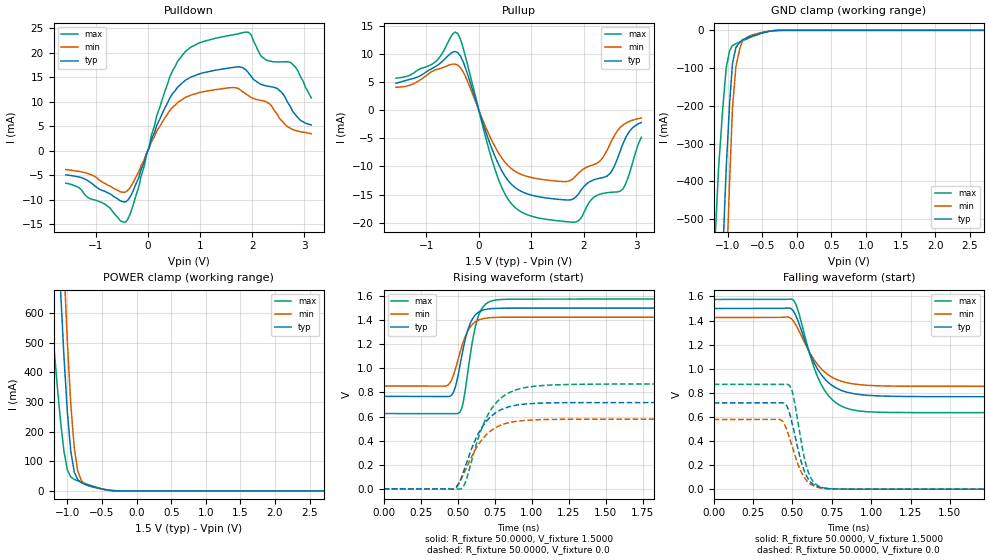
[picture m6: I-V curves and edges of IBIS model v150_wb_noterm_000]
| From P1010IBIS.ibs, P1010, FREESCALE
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[Model] v150_wb_noterm_000
|   Model v150_wb_noterm_000
| This model was characterised for following simulation conditions:
| External (pad) voltage:
|   - Typ: 1.5V,   - Min: 1.425V,   - Max: 1.575V
| Library cells for typ/min/max conditions are connected as defined below:
|  chip_pad - External Pad
|  ipp_do - Core Input
|  ipp_obe - Output Buffer Enable
|  esd_boost - vdd_io
|  gnd_io - gnd_io
|  vdd_d - vdd_d
|  vdd_io - vdd_io
|  vipp_dse_0 - gnd_io
|  vipp_dse_1 - vdd_d vdd_d gnd_io
|  vipp_dse_2 - vdd_d gnd_io gnd_io
|  vipp_dse_3 - gnd_io
|  vipp_dse_4 - gnd_io
|  vipp_dse_5 - vdd_d vdd_d gnd_io
|  vipp_dse_6 - vdd_d gnd_io vdd_d
|  vipp_dse_7 - gnd_io gnd_io vdd_d
|  vsel_0 - gnd_io
|  vsel_1 - vdd_d
| All other pins connected to ground
Model_type I/O
Polarity   Non-Inverting
Enable   Active-High
Vinl =   0.5750V
Vinh =   0.9250V
Vmeas =  0.7500V
Cref =   0.0F
Rref =   50.0000
Vref =   0.7500V
C_comp   2.2026pF   1.9235pF   2.5884pF
[Receiver Thresholds]
Vth   =  0.750V
Vinh_ac  =  0.175V
Vinh_dc  =  0.100V
Vinl_ac  = -0.175V
Vinl_dc  = -0.100V
[Temperature Range]   65.0000   0.1250k   -40.0000
[Voltage Range]   1.5000V   1.4250V   1.5750V
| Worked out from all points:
|   slope of the pulldown table from 0 to 0.225 V, typ, clamps not added: 35.6 ohm
|   slope of the pullup table from 0 to 0.225 V, typ, clamps not added: 36 ohm
|   GND clamp passes 1 mA (typ) near -0.34 V on its own axis
|   POWER clamp passes 1 mA (typ) near -0.33 V on its own axis
|   rising waveform, R_fixture 50.0000, V_fixture 1.5000: 20-80 % time 80.4ps typ, 90.1ps min, 76.9ps max; typ from 0.768 V to 1.5 V
|   rising waveform, R_fixture 50.0000, V_fixture 0.0: 20-80 % time 163ps typ, 168ps min, 166ps max; typ from 0 V to 0.716 V
|   falling waveform, R_fixture 50.0000, V_fixture 1.5000: 20-80 % time 159ps typ, 167ps min, 147ps max; typ from 1.5 V to 0.768 V
|   falling waveform, R_fixture 50.0000, V_fixture 0.0: 20-80 % time 84.1ps typ, 94.6ps min, 75.3ps max; typ from 0.716 V to 0 V
[Pulldown]
|Voltage   I(typ)   I(min)   I(max)
-1.57V    -4.914mA   -3.818mA   -6.602mA
-420mV    -10.4mA    -8.389mA   -14.49mA
-170mV    -5.399mA   -4.253mA   -7.279mA
170mV     5.137mA    3.982mA    7.064mA
420mV     10.71mA    8.187mA    14.99mA
720mV     14.36mA    10.86mA    20.23mA
1.02V     15.75mA    11.92mA    22.08mA
1.93V     15.84mA    11.19mA    24.11mA
2.23V     13.31mA    10.14mA    18.77mA
2.58V     11.69mA    5.94mA     18.1mA
2.83V     7.3mA      4.13mA     17.02mA
3.13V     5.25mA     3.46mA     10.78mA
[Pullup]
|Voltage   I(typ)   I(min)   I(max)
-1.58V    4.77mA     4.06mA     5.65mA
-850mV    7.598mA    7.066mA    8.413mA
-400mV    10.21mA    7.977mA    13.59mA
200mV     -5.632mA   -4.457mA   -7.203mA
450mV     -10.97mA   -8.649mA   -13.99mA
700mV     -13.82mA   -10.92mA   -17.37mA
1.1V      -15.32mA   -12.16mA   -19.08mA
1.8V      -15.81mA   -12.17mA   -19.92mA
2.2V      -12.37mA   -9.661mA   -15.45mA
2.5V      -11.3mA    -6.103mA   -14.62mA
2.7V      -7.204mA   -3.069mA   -14.39mA
3.1V      -2.206mA   -1.416mA   -4.843mA
[GND_clamp]
|Voltage   I(typ)   I(min)   I(max)
-1.57V    -3.686A    -4.628A    -2.289A
-1.18V    -1.14A     -1.631A    -547.3mA
-1.07V    -591.3mA   -949.6mA   -206.5mA
-1.02V    -363.2mA   -649mA     -98.9mA
-970mV    -189.9mA   -394.5mA   -53.16mA
-930mV    -87.97mA   -206.4mA   -40.43mA
-880mV    -45.34mA   -95.48mA   -35.2mA
-820mV    -30.5mA    -45.5mA    -31.02mA
-780mV    -24.31mA   -26.3mA    -27.01mA
-630mV    -13.83mA   -11.34mA   -15.55mA
-280mV    -342.7uA   -313.2uA   -187.5uA
3.13V     0A         0A         0A
[POWER_clamp]
|Voltage   I(typ)   I(min)   I(max)
-1.55V    3.265A     4.168A     1.597A
-1.25V    1.489A     2.054A     650.9mA
-1.15V    939.9mA    1.38A      364.8mA
-1.1V     686mA      1.062A     238.2mA
-1.05V    456.4mA    765.7mA    134.7mA
-1V       265.4mA    502.8mA    70.73mA
-950mV    132.2mA    289.8mA    46.77mA
-900mV    63.55mA    144.2mA    39.01mA
-850mV    37.51mA    67.07mA    34.23mA
-800mV    27.92mA    35.1mA     29.86mA
-450mV    4.486mA    4.46mA     3.638mA
3.15V     0A         0A         0A
[Ramp]
| variable   typ   min   max
dV/dt_r  0.4296/0.1627n   0.3469/0.1682n   0.5223/0.1662n
dV/dt_f  0.4395/0.1588n   0.3427/0.1668n   0.5638/0.1473n
R_load = 50.0000
[Rising Waveform]
R_fixture= 50.0000
V_fixture= 1.5000
V_fixture_min= 1.4250
V_fixture_max= 1.5750
|time   V(typ)   V(min)   V(max)
0s        767.5mV    853.8mV    624.9mV
422.9ps   766.6mV    853.9mV    624.9mV
475.2ps   811.9mV    955.6mV    624.7mV
512.4ps   1.002V     1.116V     633.6mV
536.5ps   1.157V     1.215V     711.5mV
569.9ps   1.324V     1.314V     981.3mV
629.7ps   1.456V     1.394V     1.395V
685.2ps   1.488V     1.416V     1.529V
754.7ps   1.498V     1.423V     1.567V
5ns       1.5V       1.425V     1.575V
[Rising Waveform]
R_fixture= 50.0000
V_fixture= 0.0
V_fixture_min= 0.0
V_fixture_max= 0.0
|time   V(typ)   V(min)   V(max)
0s        7.324uV    39.66uV    145.2nV
471.2ps   -1.638mV   2.095mV    195.8uV
499.2ps   24.09mV    30.35mV    -1.051mV
525.6ps   93.62mV    85.45mV    1.76mV
559.4ps   213.2mV    174.8mV    79.48mV
640.1ps   460mV      366.7mV    425mV
730.7ps   606.6mV    487.4mV    667.9mV
838.2ps   678mV      546.9mV    791.8mV
986.6ps   707mV      571mV      847mV
5ns       716.1mV    578.2mV    870.5mV
[Falling Waveform]
R_fixture= 50.0000
V_fixture= 1.5000
V_fixture_min= 1.4250
V_fixture_max= 1.5750
|time   V(typ)   V(min)   V(max)
0s        1.5V       1.425V     1.575V
466.9ps   1.504V     1.429V     1.575V
503.3ps   1.483V     1.4V       1.572V
535.8ps   1.393V     1.328V     1.48V
606.2ps   1.139V     1.141V     1.135V
638.3ps   1.047V     1.072V     1.004V
706ps     913.6mV    971.4mV    816.5mV
801.2ps   824.9mV    900mV      695.7mV
925ps     785.4mV    867.4mV    648.7mV
5ns       767.5mV    853.8mV    635.4mV
[Falling Waveform]
R_fixture= 50.0000
V_fixture= 0.0
V_fixture_min= 0.0
V_fixture_max= 0.0
|time   V(typ)   V(min)   V(max)
0s        716.1mV    578.2mV    870.5mV
419.7ps   716.3mV    578.5mV    870.5mV
452.8ps   709.3mV    528.9mV    870.8mV
478.9ps   641.6mV    433.7mV    862.2mV
505.8ps   502.6mV    321.9mV    771.6mV
556.1ps   223.7mV    140.8mV    389mV
603.6ps   78.76mV    52.66mV    130.8mV
655.1ps   23.25mV    17.34mV    34.05mV
724.9ps   4.453mV    3.884mV    5.351mV
5ns       7.702uV    39.93uV    332.6nV
